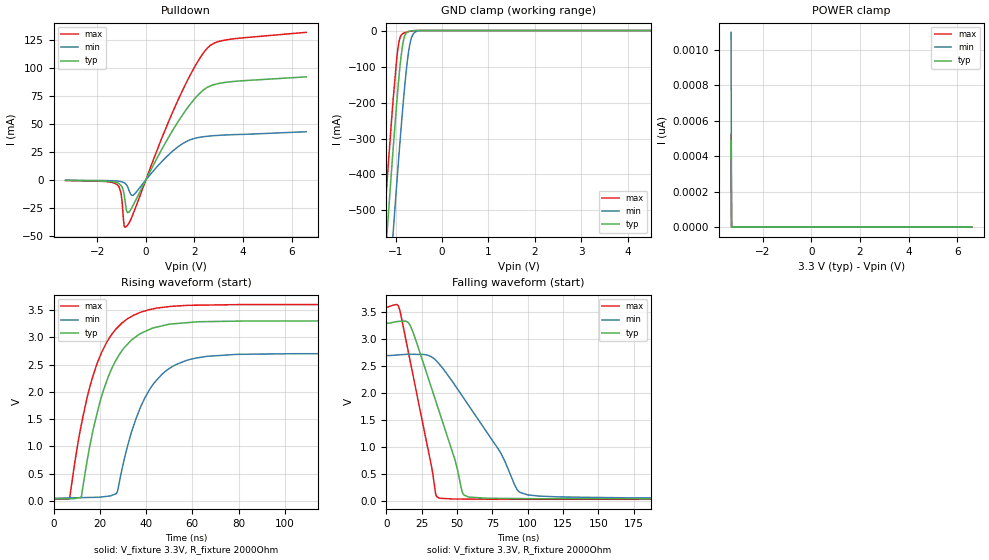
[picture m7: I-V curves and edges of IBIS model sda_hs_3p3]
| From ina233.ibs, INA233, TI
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|   sda_hs_3p3
[Model]   sda_hs_3p3
Model_type   I/O_open_drain
Polarity   Non-Inverting
Vinl = 0.4
Vinh = 2.31
Vmeas = 1.65
Vref = 3.3
Cref = 2pF
Rref = 2000
|   typ   min   max
C_comp   1.203E-12   1.196E-12  1.271E-12
|C_comp_pull_down   1.360E-12   1.339E-12   1.374E-12
| Where Nom  PVT is Nominal Process, 3.3V, 25C
|   Fast PVT is Strong Process,  3.6V, -40C
|   Slow PVT is Weak Process,   2.7V, 125C
[Voltage Range]   3.3   2.7   3.6
[Temperature Range]   25   125   -40
[Pullup Reference]   3.3   2.7   3.6
[Pulldown Reference]   0   0   0
[Power Clamp Reference]   3.3   2.7   3.6
[GND Clamp Reference]   0   0   0
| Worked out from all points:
|   slope of the pulldown table from 0 to 0.495 V, typ, clamps not added: 23.7 ohm
|   GND clamp passes 1 mA (typ) near -0.67 V on its own axis
|   falling waveform, V_fixture 3.3V, R_fixture 2000Ohm: 20-80 % time 24.2ns typ, 38.4ns min, 16.5ns max; typ from 3.3 V to 0.039 V
|   rising waveform, V_fixture 3.3V, R_fixture 2000Ohm: 20-80 % time 13.6ns typ, 14ns min, 13.4ns max; typ from 0.039 V to 3.3 V
[Pulldown]
|   Voltage   I(typ)   I(min)   I(max)
-3.3V     -277.8uA   -132.7uA   -350.1uA
-1.191V   -2.338mA   -871.4uA   -3.896mA
-1.033V   -4.45mA    -1.339mA   -10.36mA
-983.4mV  -5.979mA   -1.591mA   -17.46mA
-894.3mV  -12.41mA   -2.333mA   -39.9mA
-815.1mV  -24.49mA   -3.669mA   -41.95mA
-745.8mV  -29.08mA   -6.081mA   -40.22mA
-508.2mV  -21.97mA   -13.35mA   -29.54mA
1.264V    49.95mA    28.7mA     68.48mA
2.511V    82.59mA    39.12mA    117.5mA
3.343V    87.49mA    40.35mA    125.4mA
6.6V      92.24mA    43.2mA     132mA
[GND Clamp]
|   Voltage   I(typ)   I(min)   I(max)
-3.3V     -4.686A    -4.907A    -4.556A
-1.29V    -760.6mA   -998mA     -618.3mA
-1.251V   -686.8mA   -924.1mA   -544.4mA
-1.181V   -559mA     -795.9mA   -417mA
-1.053V   -329.6mA   -562.7mA   -192.6mA
-973.5mV  -198.4mA   -424.1mA   -76.5mA
-924mV    -124.9mA   -340.5mA   -29.61mA
-815.1mV  -19.77mA   -171.5mA   -6.69mA
-735.9mV  -3.683mA   -74.37mA   -3.342mA
-676.5mV  -1.199mA   -28.91mA   -1.665mA
-508.2mV  -32.1uA    -958.7uA   -51.41uA
6.6V      0A         0A         0A
[POWER Clamp]
|   Voltage   I(typ)   I(min)   I(max)
-3.3V     486.6pA    1.097nA    522.5pA
-3.28V    0A         0A         0A
-3.27V    0A         0A         0A
6.6V      0A         0A         0A
[Ramp]
R_load = 2000
|   typ   min   max
dV/dt_r   1.95658/1.35731e-08   1.58967/1.40363e-08   2.14084/1.33913e-08
dV/dt_f   1.95658/2.42376e-08   1.58967/3.84501e-08   2.14084/1.65502e-08
[Falling Waveform]
V_fixture = 3.3V
V_fixture_min = 2.7V
V_fixture_max = 3.6V
R_fixture = 2000Ohm
C_fixture = 0F
|   Time   V(typ)   V(min)   V(max)
0s        3.3V       2.7V       3.6V
9.384ns   3.33V      2.71V      3.553V
17.34ns   3.232V     2.72V      2.538V
34.92ns   1.861V     2.613V     137.7mV
37.39ns   1.662V     2.541V     55.46mV
55.16ns   109.4mV    1.892V     37.07mV
80.86ns   49.36mV    895.9mV    33.33mV
92.38ns   46.56mV    218.3mV    33.29mV
99.63ns   44.81mV    117.3mV    33.27mV
500ns     39.03mV    50.55mV    31.92mV
[Rising Waveform]
V_fixture = 3.3V
V_fixture_min = 2.7V
V_fixture_max = 3.6V
R_fixture = 2000Ohm
C_fixture = 0F
|   Time   V(typ)   V(min)   V(max)
0s        39.03mV    50.55mV    31.92mV
6.922ns   43.69mV    57.64mV    39.74mV
11.97ns   66.98mV    62.81mV    1.385V
19.77ns   1.768V     70.81mV    2.618V
27.25ns   2.598V     140.6mV    3.163V
35.91ns   3.018V     1.536V     3.427V
44.76ns   3.188V     2.222V     3.535V
57.23ns   3.265V     2.572V     3.583V
79.08ns   3.295V     2.687V     3.597V
500ns     3.3V       2.7V       3.6V
